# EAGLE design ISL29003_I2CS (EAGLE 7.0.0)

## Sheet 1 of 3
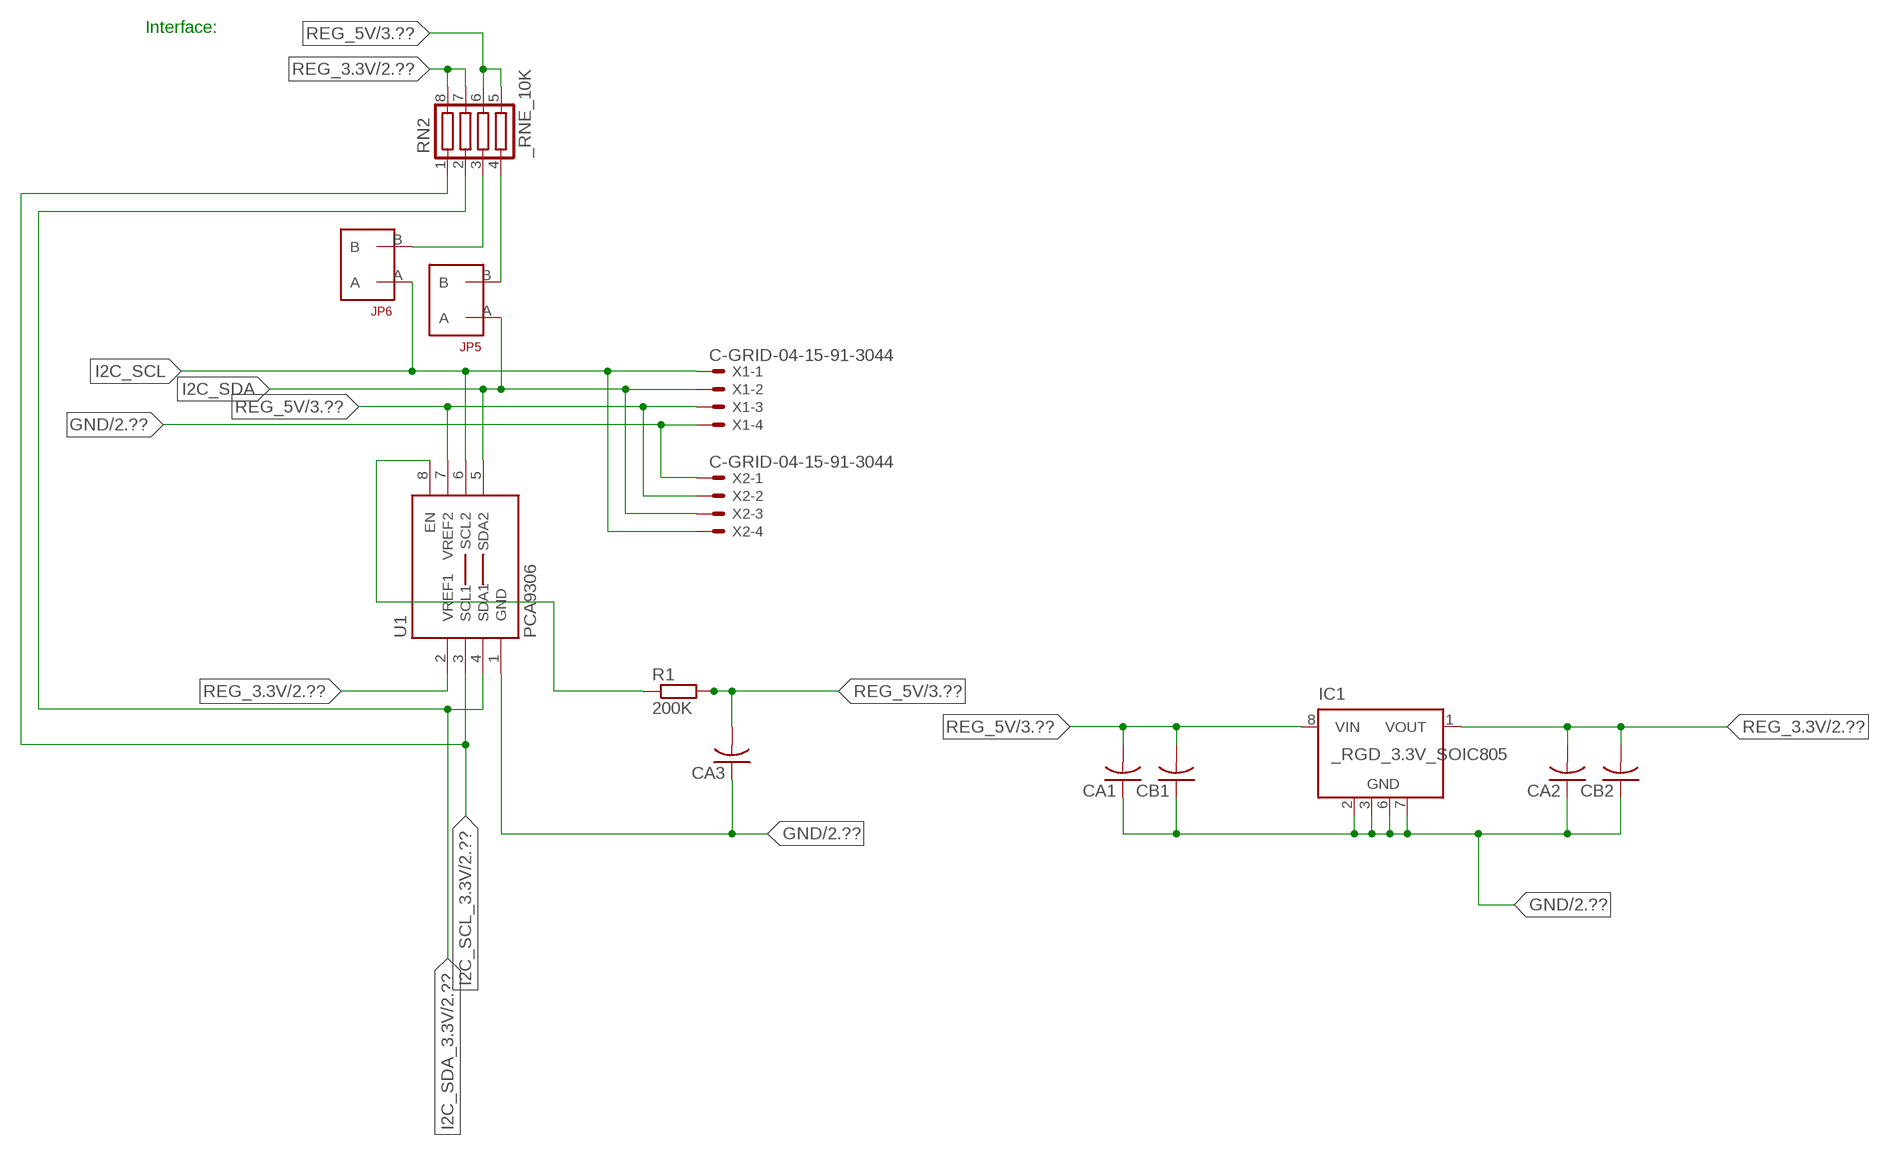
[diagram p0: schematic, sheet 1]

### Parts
CA1  CC1206KRX7R9BB104  [.1UF]
CA2  CC1206KRX7R9BB104  [.1UF]
CA3  CC1206KRX7R9BB104  [.1UF]
CB1  TMK316F106ZL-TC1206K  [TMK316F106ZL-T]
CB2  TMK316F106ZL-TC1206K  [TMK316F106ZL-T]
IC1  _RGD_3.3V_SOIC805  [_RGC_3.3V_SOIC8]
JP5  JUMPER_1X2_2MM  [JUMPER_1X2_2MM]
JP6  JUMPER_1X2_2MM  [JUMPER_1X2_2MM]
R1  200K  RESISTOR_SMT-0603  [R603]
RN2  _RNE_10K  [RNE]
U1  PCA9306  PCA9306_NCD  [PSOP-8]
X1  C-GRID-04-15-91-3044  [15-91-04]
X2  C-GRID-04-15-91-3044  [15-91-04]

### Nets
GND: CA1.1 CA2.1 CA3.1 CB1.1 CB2.1 IC1.2(GND) IC1.3(GND) IC1.6(GND) IC1.7(GND) U1.1(GND) X1.4 X2.1 ; also sheet 2,3
I2C_SCL: JP6.A U1.6(SCL2) X1.1 X2.4
I2C_SCL_3.3V: RN2.1 U1.3(SCL1) ; also sheet 2
I2C_SDA: JP5.A U1.5(SDA2) X1.2 X2.3
I2C_SDA_3.3V: RN2.2 U1.4(SDA1) ; also sheet 2
N$1: JP6.B RN2.3
N$2: JP5.B RN2.4
N$24: R1.1 U1.8(EN)
REG_3.3V: CA2.2 CB2.2 IC1.1(VOUT) RN2.7 RN2.8 U1.2(VREF1) ; also sheet 2
REG_5V: CA1.2 CA3.2 CB1.2 IC1.8(VIN) R1.2 RN2.5 RN2.6 U1.7(VREF2) X1.3 X2.2 ; also sheet 3
Unconnected: IC1.4(NC) IC1.5(NC)

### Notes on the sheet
- Interface:

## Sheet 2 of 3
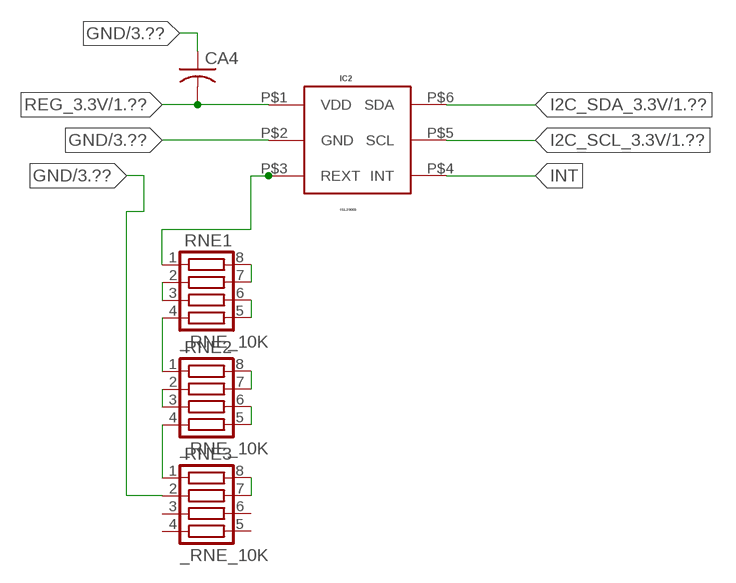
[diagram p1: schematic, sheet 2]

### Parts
CA4  _CA_.10UF_50VC1206K  [_CA_.1UF_50V]
IC2  ISL29003  [ODFN6]
RNE1  _RNE_10K  [RNE]
RNE2  _RNE_10K  [RNE]
RNE3  _RNE_10K  [RNE]

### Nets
GND: CA4.1 IC2.P$2(GND) RNE3.2 ; also sheet 1,3
I2C_SCL_3.3V: IC2.P$5(SCL) ; also sheet 1
I2C_SDA_3.3V: IC2.P$6(SDA) ; also sheet 1
INT: IC2.P$4(INT)
N$5: IC2.P$3(REXT) RNE1.1
N$214: RNE1.7 RNE1.8
N$215: RNE1.2 RNE1.3
N$216: RNE1.5 RNE1.6
N$217: RNE1.4 RNE2.1
N$218: RNE2.7 RNE2.8
N$219: RNE2.2 RNE2.3
N$220: RNE2.5 RNE2.6
N$221: RNE2.4 RNE3.1
N$222: RNE3.7 RNE3.8
REG_3.3V: CA4.2 IC2.P$1(VDD) ; also sheet 1
Unconnected: RNE3.3 RNE3.4 RNE3.5 RNE3.6

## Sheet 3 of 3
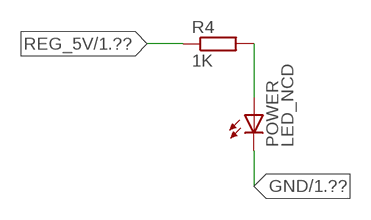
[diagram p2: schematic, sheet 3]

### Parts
POWER  LED_NCD  [CHIPLED_0603]
R4  1K  RESISTOR_SMT-0402  [R402]

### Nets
GND: POWER.C ; also sheet 1,2
N$4: POWER.A R4.2
REG_5V: R4.1 ; also sheet 1

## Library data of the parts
CA1-CA3 = NCD_ULTIMATE_LIBRARY:CC1206KRX7R9BB104: Capacitor CA .1uF 50V SMT C1206K CC1206KRX7R9BB104
CA4 = NCD_ULTIMATE_LIBRARY:_CA_.10UF_50V: Capacitor .1uF SMT
CB1 CB2 = NCD_ULTIMATE_LIBRARY:TMK316F106ZL-T: Capacitor CB 10uF SMT 1206 TMK316F106ZL-T
IC1 = NCD_ULTIMATE_LIBRARY:_RGD_3.3V_SOIC8: Regulator Linear 3.3V Chip Positive VOLTAGE REGULATOR Digikey 497-1199-2-ND/L78L33ACD13TR
IC2 = NCD_ULTIMATE_bhaskar:ISL29003: Digikey ISL29003IROZ-T7DKR-ND/ISL29003IROZ-T7
JP5 JP6 = NCD_ULTIMATE_CONNECTORS:JUMPER_1X2_2MM
POWER = NCD_ULTIMATE_LIBRARY:LED_NCD: LED Digikey 754-1132-2-ND/APT2012SRCPRV
R1 R4 = NCD_ULTIMATE_LIBRARY:RESISTOR_SMT: NCD Resistor
RN2 RNE1-RNE3 = NCD_ULTIMATE_LIBRARY:_RNE_10K: Resistor Array RNE SMT 10K x 4 Single Resistor Source: http://www.ctscorp.com/components/Datasheets/CTSChipArrayDs.pdf Digikey 742C083103JPTR-ND/742C083103JP; OC_FARNELL: unknown; OC_NEWARK: unknown
U1 = NCD_ULTIMATE_LIBRARY:PCA9306_NCD: NCD Bidirectional I2C level shifter. NOT compatible with all available part number pinout schemes- DOUBLE CHECK!!!; PROD_ID: IC-10023
X1 X2 = NCD_ULTIMATE_CONNECTORS:C-GRID-04: CONNECTOR 4-Pos I2C wire to board 2.54 mm (0.100") pitch header Digikey WM1342-ND/0015912045; OC_FARNELL: unknown; OC_NEWARK: unknown

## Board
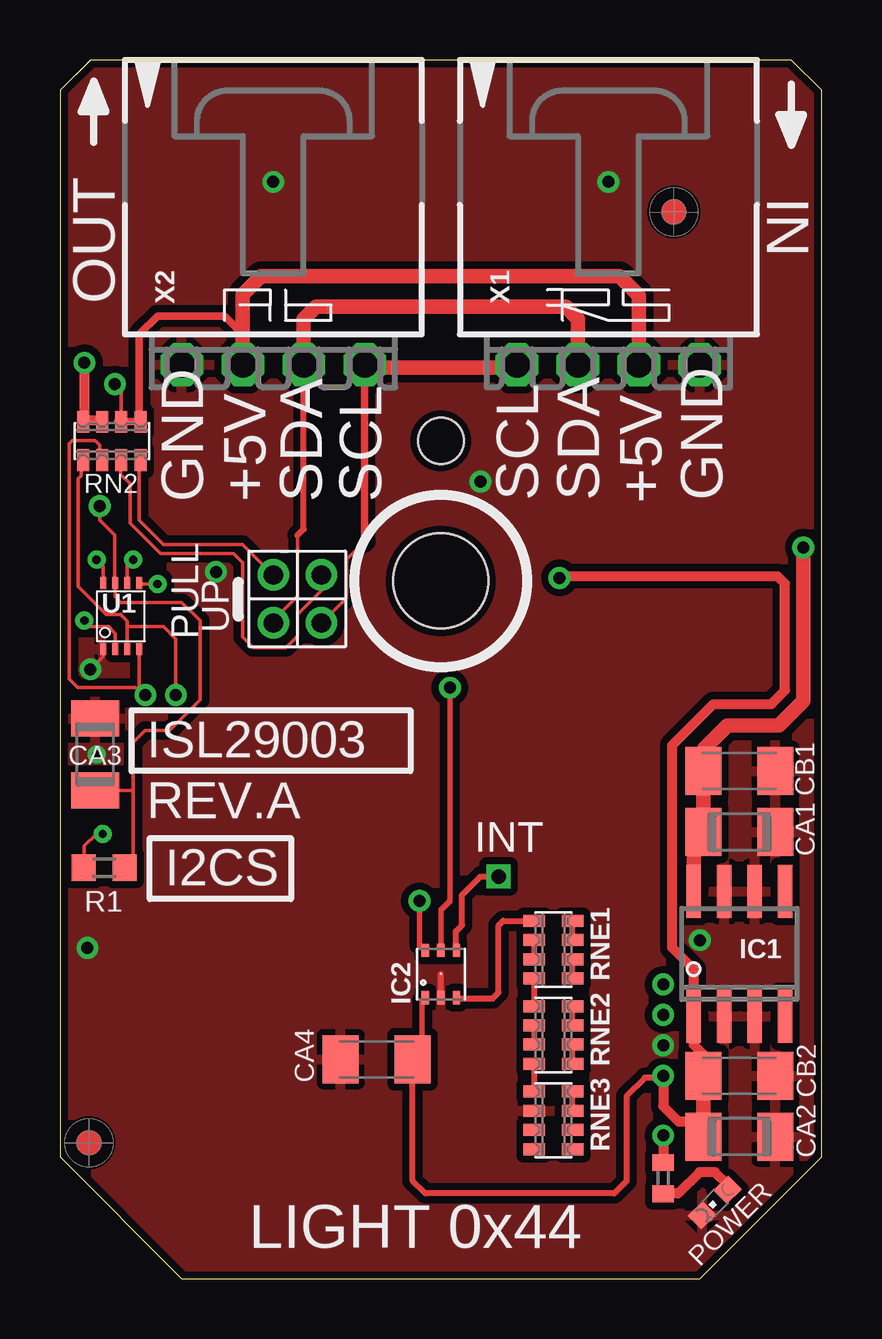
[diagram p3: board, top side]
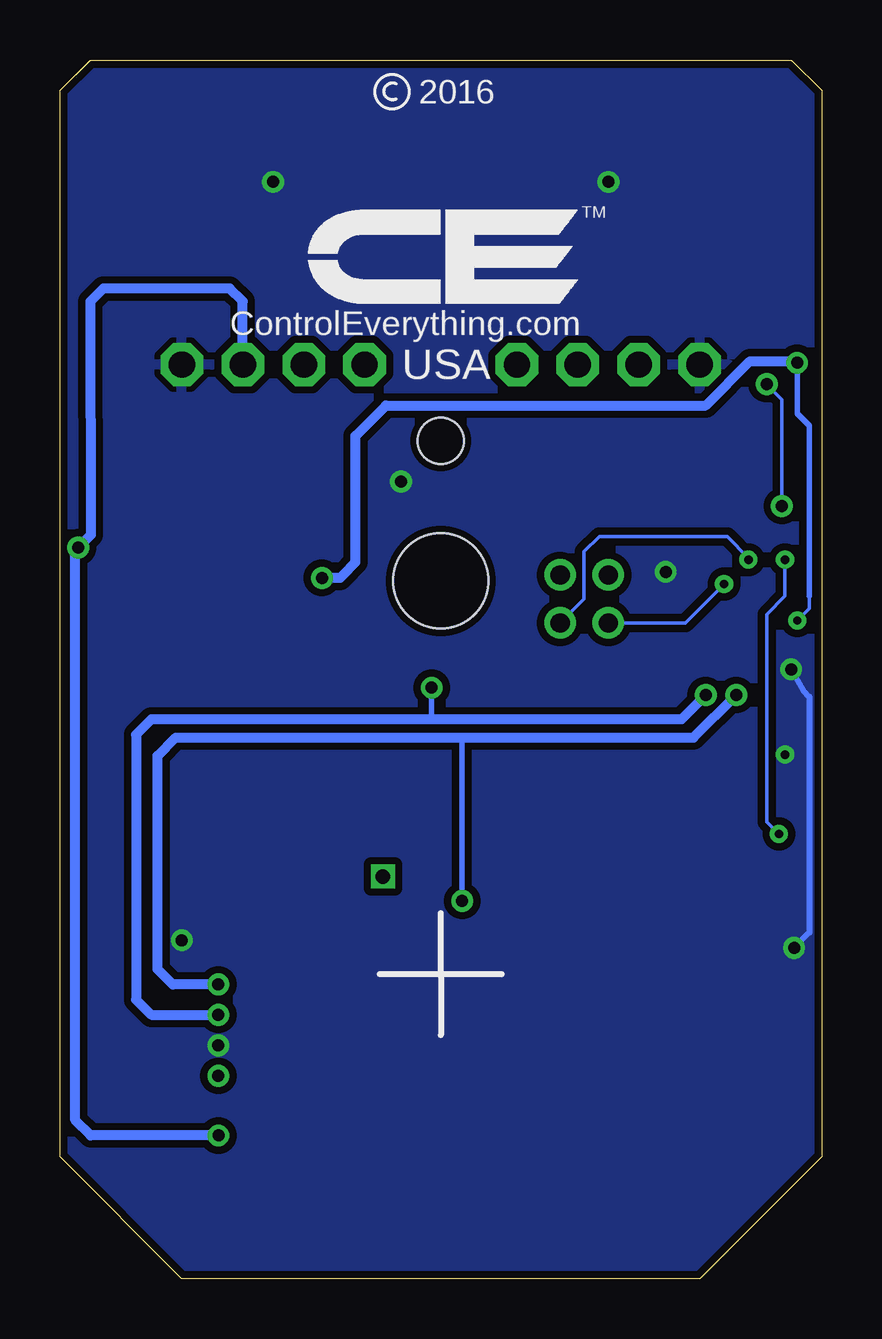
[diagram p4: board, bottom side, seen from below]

Size 31.75 x 50.8 mm. Coordinates in mm from the lower left corner, seen from the top.
Outline: 31.75,5.08 31.75,49.53 30.48,50.8 1.27,50.8 0,49.53 0,5.08 5.08,0 26.67,0 31.75,5.08
Outline: 31.75,5.08 31.75,49.53 30.48,50.8 1.27,50.8 0,49.53 0,5.08 5.08,0 26.67,0 31.75,5.08
Copper layers (1*16): Top 0.035mm / dielectric 1.5mm / Bottom 0.035mm
Design rules "default": minimum track width 5mil, minimum drill 24mil, track to track 5mil, track to pad 5mil, pad to pad 5mil, via to via 5mil, smd to smd 5mil, copper to edge 10mil, drill to drill 8mil, minimum pad ring 10mil, minimum via ring 8mil, stop-mask expansion 2mil, vias tented up to drill 0mil, thermal gap 10mil
Holes 3.96 mm at 15.88,29.08
Holes 1.91 mm at 15.88,34.93

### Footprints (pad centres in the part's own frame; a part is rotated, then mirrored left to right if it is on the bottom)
.1UF = smd 1.5 x 2: 1 -1.5,0; 2 1.5,0
_CA_.1UF_50V = smd 1.5 x 2: 1 -1.5,0; 2 1.5,0
TMK316F106ZL-T = smd 1.5 x 2: 1 -1.5,0; 2 1.5,0
_RGC_3.3V_SOIC8 = smd 0.6 x 2.2: 1 -1.905,-2.6; 2 -0.635,-2.6; 3 0.635,-2.6; 4 1.905,-2.6; 5 1.905,2.6; 6 0.635,2.6; 7 -0.635,2.6; 8 -1.905,2.6
ODFN6 = smd 0.55 x 0.3: P$1 -0.98,0.65; P$2 -0.98,0; P$3 -0.98,-0.65; P$4 0.98,-0.65; P$5 0.98,0; P$6 0.98,0.65
JUMPER_1X2_2MM = drill 0.8: A 0,2; B 0,0
CHIPLED_0603 = smd 0.8 x 0.876: A 0,-0.75; C 0,0.75
R603 = smd 1 x 1.1: 1 -0.85,0; 2 0.85,0
R402 = smd 0.7 x 0.9: 1 -0.65,0; 2 0.65,0
RNE = smd 0.5 x 0.9: 1 -1.2,-0.8; 2 -0.4,-0.8; 3 0.4,-0.8; 4 1.2,-0.8; 5 1.2,0.8; 6 0.4,0.8; 7 -0.4,0.8; 8 -1.2,0.8
PSOP-8 = smd 0.25 x 0.5: 1 -0.73,-1.37; 2 -0.23,-1.37; 3 0.27,-1.37; 4 0.77,-1.37; 5 0.77,1.38; 6 0.27,1.38; 7 -0.23,1.38; 8 -0.73,1.38
15-91-04 = drill 1.1 pad 1.778 octagon: 1 -3.81,-7.62; 2 -1.27,-7.62; 3 1.27,-7.62; 4 3.81,-7.62

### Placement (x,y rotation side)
CA1  28.32,18.62 180 top
CA2  28.32,5.92 180 top
CA3  1.46,21.86 270 top
CA4  13.21,9.14 0 top
CB1  28.32,21.16 180 top
CB2  28.32,8.46 180 top
IC1  28.32,13.54 0 top
IC2  15.88,12.7 90 top
JP5  8.89,29.34 180 top
JP6  10.9,29.34 180 top
POWER  27.3,3.18 135 top
R1  1.84,17.13 0 top
R4  25.15,4.19 270 top
RN2  2.16,34.93 0 top
RNE1  20.57,13.72 270 top
RNE2  20.57,10.16 270 top
RNE3  20.57,6.6 270 top
U1  2.54,27.61 0 top
U$5  [VISION_REF10]  1.21,5.66 90 top
U$28  [VISION_REF10]  25.59,44.46 90 top
X1  22.86,45.72 0 top
X2  8.89,45.72 0 top

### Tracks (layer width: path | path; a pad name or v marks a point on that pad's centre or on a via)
GND  (via drill 0.35, 0.5)
  Top 0.152: CA3.1 1.52,23.42 1.52,23.62 | v1.27,25.4 1.81,25.94 U1.1
  Top 0.254: IC2.P$2 15.88,12.7
  Bottom 0.254: v1.27,25.4 0.76,24.51 0.51,24.26 0.51,14.43 v1.15,13.79
  other vias: 8.89,45.72 22.86,45.72 25.15,9.73 17.53,33.22 26.67,14.11 6.5,29.46 1.52,21.84
  pour Bottom (isolate 0.305): -0.64,5.08 -0.64,49.53 1.27,51.44 30.48,51.44 32.38,49.53 32.38,5.08 26.67,-0.63 5.08,-0.63
  pour Top (isolate 0.305): 4.45,-1.27 -1.27,4.45 -1.27,50.17 0.64,52.07 31.11,52.07 33.02,50.17 33.02,4.45 27.3,-1.27
I2C_SCL  (via drill 0.35)
  Top 0.152: 12.7,30.73 11.94,29.97 11.94,28.38 JP6.A | v3.05,29.97 2.81,29.73 U1.6
  Top 0.305: 12.7,30.73 X2.4
  Top 0.406: X2.4 12.7,37.97 | 19.05,37.97 X1.1
  Top 0.61: 12.7,37.97 19.05,37.97
  Bottom 0.152: JP6.A 9.91,28.33 9.91,30.3 9.27,30.94 3.94,30.94 3.05,30.05 v3.05,29.97
I2C_SCL_3.3V  (via drill 0.5)
  Top 0.152: RN2.1 0.89,34.07 0.89,33.48 0.77,33.35 0.77,28.84 1.92,27.69 2.54,27.69 2.81,27.42 2.81,27.18 | 2.81,27.18 U1.3 | v4.83,24.33 v4.83,24.34 4.83,26.67 4.32,27.18 2.81,27.18
  Top 0.229: IC2.P$5 15.88,15.37 16.26,15.75 v16.26,24.64
  Bottom 0.229: v16.26,24.64 16.26,23.32
  Bottom 0.406: v4.83,24.33 5.84,23.32 16.26,23.32 27.94,23.32 28.58,22.68 28.58,11.63 27.94,11 v25.15,11
I2C_SDA  (via drill 0.35)
  Top 0.152: JP5.A 8.89,27.44 9.91,28.45 9.91,30.99 | U1.5 3.34,28.96 v4.06,28.96
  Top 0.254: 9.91,30.99 10.16,31.25 X2.3
  Top 0.61: X2.3 10.16,40.01 10.67,40.51 21.09,40.51 21.59,40.01 X1.2
  Bottom 0.152: v4.06,28.96 5.68,27.34 JP5.A
I2C_SDA_3.3V  (via drill 0.5)
  Top 0.152: RN2.2 1.65,34.14 1.65,34.75 1.46,34.94 0.51,34.94 0.38,34.81 0.38,26.37 0.38,26.36 0.38,24.99 0.74,24.64 3.15,24.64 3.45,24.33 v3.56,24.33 3.31,24.58 U1.4
  Top 0.229: IC2.P$6 14.99,13.92 v14.99,15.75
  Bottom 0.229: v14.99,15.75 14.99,22.56
  Bottom 0.406: v25.15,12.27 27.05,12.27 27.69,12.9 27.69,21.79 26.93,22.56 14.99,22.56 5.34,22.56 v3.56,24.33
INT  (via drill 0.6)
  Top 0.254: IC2.P$4 16.51,14.48 16.76,14.73 16.76,16 17.53,16.76 v18.29,16.76
N$1
  Top 0.152: JP6.B 10.92,29.31 10.92,28.7 9.91,27.69 9.91,26.8 9.42,26.31 8.06,26.31 7.62,26.75 7.62,29.84 7.24,30.23 4.19,30.23 2.92,31.5 2.92,33.15 2.54,33.53 2.54,34.1 RN2.3
  Top 0.305: 2.54,34.02 RN2.3
N$2
  Top 0.152: JP5.B 7.62,30.61 4.32,30.61 3.3,31.62 3.3,34.07 RN2.4
  Top 0.305: 3.37,33.88 RN2.4
N$4
  Top 0.406: POWER.A 27.84,3.92 27.3,4.45 26.67,4.45 25.78,3.56 25.16,3.56 R4.2
N$5
  Top 0.254: IC2.P$3 16.56,11.68 18.03,11.68 18.29,11.94 18.29,14.73 18.47,14.92 RNE1.1
N$24  (via drill 0.35)
  Top 0.152: R1.1 1.02,17.16 1.02,18.03 1.52,18.54 v1.78,18.54 | v1.52,29.97 1.81,29.69 U1.8
  Bottom 0.152: v1.78,18.54 2.29,19.05 2.29,27.69 1.52,28.45 v1.52,29.97
N$214
  Top 0.254: RNE1.7 RNE1.8
N$215
  Top 0.254: RNE1.3 RNE1.2
N$216
  Top 0.254: RNE1.5 RNE1.6
N$217
  Top 0.254: RNE2.1 RNE1.4
N$218
  Top 0.254: RNE2.7 RNE2.8
N$219
  Top 0.254: RNE2.3 RNE2.2
N$220
  Top 0.254: RNE2.5 RNE2.6
N$221
  Top 0.254: RNE3.1 RNE2.4
N$222
  Top 0.254: RNE3.7 RNE3.8
REG_3.3V  (via drill 0.35, 0.5)
  Top 0.152: v1.02,27.43 1.27,27.18 2.03,27.18 2.31,26.9 U1.2
  Top 0.229: IC2.P$1 15.09,11.58 15.09,9.52 CA4.2
  Top 0.254: v25.15,8.46 25.07,8.38 24.38,8.38 23.62,7.62 23.62,4.06 23.11,3.56 15.24,3.56 14.71,4.09 CA4.2
  Top 0.406: CB2.2 26.82,9.35 26.42,9.75 26.42,10.36 | v25.15,8.46 25.15,7.19 25.78,6.55 26.82,6.55 | IC1.1 26.42,12.9 25.53,13.79 25.53,22.24 27.24,23.95 29.66,23.95 30.23,24.52 30.23,28.97 29.91,29.29 20.9,29.29 v20.83,29.21 | 26.52,5.62 CA2.2 | v1.02,38.18 1.02,35.78 | 1.02,35.78 RN2.8 | 1.02,35.78 1.71,35.78 RN2.7
  Top 0.61: CB2.2 26.82,6.55 CA2.2 | 26.42,10.36 IC1.1
  Bottom 0.152: 0.51,28.45 0.51,27.94 v1.02,27.43
  Bottom 0.229: 0.51,28.45 0.51,35.56 1.02,36.07 v1.02,38.18
  Bottom 0.406: v1.02,38.18 1.08,38.24 2.99,38.24 4.83,36.4 18.16,36.4 19.43,35.13 19.43,29.87 19.94,29.34 20.07,29.21 v20.83,29.21
REG_5V  (via drill 0.5)
  Top 0.152: RN2.6 2.56,37.01 v2.29,37.29 | R1.2 3.05,17.49 3.05,20.36 | 3.05,20.36 3.05,22.35 3.56,22.86 4.57,22.86 5.84,24.13 5.84,27.43 5.08,28.19 2.54,28.19 2.31,28.43 U1.7 2.29,29.01 2.29,30.99 1.65,31.62 v1.65,32.21 | CA3.2 3.05,20.36
  Top 0.305: 7.62,39.37 7.5,39.37 | 2.42,35.74 RN2.6 RN2.5 3.31,35.8 3.31,39.37 4.07,40.13 6.86,40.13 7.62,39.37 | X2.2 7.62,39.37
  Top 0.406: v25.15,5.97 R4.1
  Top 0.61: X2.2 7.62,41.02 8.38,41.78 23.32,41.78 24.13,40.97 X1.3 | IC1.8 26.42,18.21 CA1.2 CB1.2 26.86,21.2 26.86,22.11 27.82,23.06 29.98,23.06 30.99,24.08 v30.99,30.48
  Bottom 0.152: v1.65,32.21 1.65,36.65 v2.29,37.29
  Bottom 0.406: X1.3 24.13,40.74 24.67,41.28 29.94,41.28 30.48,40.73 30.47,31 v30.99,30.48 31.11,30.36 31.11,6.6 30.48,5.97 v25.15,5.97

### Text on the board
tPlace: LIGHT 0x44
tNames: IN | OUT | GND | +5V | SDA | SCL | SCL | SDA | +5V | GND | PULL | UP | ISL29003 | REV.A | INT | I2CS
bNames: 2016 | TM | ControlEverything.com | USA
